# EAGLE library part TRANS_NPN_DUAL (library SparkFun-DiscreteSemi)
Dual NPN Transistors in Single Package The MBT3904W1 puts two general purpose 3904 NPN transistors in a single package. Datasheet SparkFun Products: SparkFun ESP32 Thing
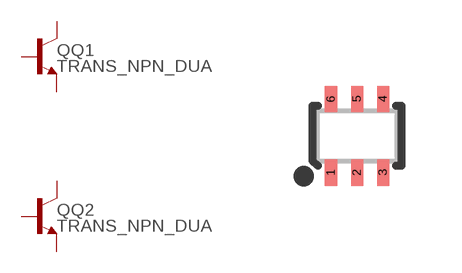
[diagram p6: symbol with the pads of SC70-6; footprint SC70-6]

Designator prefix Q; gates Q1=NPN Q2=NPN

## TRANS_NPN_DUAL-MBT3904DW1T1 (PROD_ID: TRANS-13337)  [SC70-6]
1  Q2:E  pas
2  Q2:B  pas
3  Q1:C  pas
4  Q1:E  pas
5  Q1:B  pas
6  Q2:C  pas

## Footprint SC70-6 (pad centres in mm)
SC-88/SC70-6/SOT-363 6-pin Package Example Datasheet
smd 0.3 x 0.66: 1 -0.65,-0.92; 2 0,-0.92; 3 0.65,-0.92; 4 0.65,0.92; 5 0,0.92; 6 -0.65,0.92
